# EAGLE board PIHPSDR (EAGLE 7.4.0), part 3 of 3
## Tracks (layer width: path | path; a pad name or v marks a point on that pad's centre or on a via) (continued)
N$1188  (via drill 0.8 pad 1.93) (continued)
  other vias: 151.94,107.22
N$1189  (via drill 0.8 pad 1.93)
  other vias: 151.94,104.68
N$1190  (via drill 0.8 pad 1.93)
  other vias: 151.94,102.14
N$1191  (via drill 0.8 pad 1.93)
  other vias: 151.94,99.6
N$1192  (via drill 0.8 pad 1.93)
  other vias: 151.94,97.06
N$1193  (via drill 0.8 pad 1.93)
  other vias: 151.94,94.52
N$1194  (via drill 0.8 pad 1.93)
  other vias: 151.94,91.98
N$1195  (via drill 0.8 pad 1.93)
  other vias: 151.94,89.44
N$1196  (via drill 0.8 pad 1.93)
  other vias: 151.94,86.9
N$1197  (via drill 0.8 pad 1.93)
  other vias: 151.94,84.36
N$1198  (via drill 0.8 pad 1.93)
  other vias: 151.94,81.82
N$1199  (via drill 0.8 pad 1.93)
  other vias: 151.94,79.28
N$1200  (via drill 0.8 pad 1.93)
  other vias: 151.94,76.74
N$1201  (via drill 0.8 pad 1.93)
  other vias: 151.94,74.2
N$1202  (via drill 0.8 pad 1.93)
  other vias: 151.94,71.66
N$1203  (via drill 0.8 pad 1.93)
  other vias: 151.94,69.12
N$1204  (via drill 0.8 pad 1.93)
  other vias: 151.94,66.58
N$1205  (via drill 0.8 pad 1.93)
  other vias: 151.94,64.04
N$1206  (via drill 0.8 pad 1.93)
  other vias: 151.94,61.5
N$1207  (via drill 0.8 pad 1.93)
  other vias: 151.94,58.96
N$1208  (via drill 0.8 pad 1.93)
  other vias: 151.94,56.42
N$1209  (via drill 0.8 pad 1.93)
  other vias: 151.94,53.88
N$1210  (via drill 0.8 pad 1.93)
  other vias: 151.94,51.34
N$1211  (via drill 0.8 pad 1.93)
  other vias: 151.94,48.8
N$1212  (via drill 0.8 pad 1.93)
  other vias: 151.94,46.26
N$1213  (via drill 0.8 pad 1.93)
  other vias: 151.94,43.72
N$1214  (via drill 0.8 pad 1.93)
  other vias: 151.94,41.18
N$1215  (via drill 0.8 pad 1.93)
  other vias: 151.94,38.64
N$1216  (via drill 0.8 pad 1.93)
  other vias: 151.94,36.1
N$1217  (via drill 0.8 pad 1.93)
  other vias: 151.94,33.56
N$1218  (via drill 0.8 pad 1.93)
  other vias: 151.94,31.02
N$1219  (via drill 0.8 pad 1.93)
  other vias: 151.94,28.48
N$1220  (via drill 0.8 pad 1.93)
  other vias: 151.94,25.94
N$1222  (via drill 0.8 pad 1.93)
  other vias: 154.48,119.92
N$1223  (via drill 0.8 pad 1.93)
  other vias: 154.48,117.38
N$1224  (via drill 0.8 pad 1.93)
  other vias: 154.48,114.84
N$1225  (via drill 0.8 pad 1.93)
  other vias: 154.48,112.3
N$1226  (via drill 0.8 pad 1.93)
  other vias: 154.48,109.76
N$1227  (via drill 0.8 pad 1.93)
  other vias: 154.48,107.22
N$1228  (via drill 0.8 pad 1.93)
  other vias: 154.48,104.68
N$1229  (via drill 0.8 pad 1.93)
  other vias: 154.48,102.14
N$1230  (via drill 0.8 pad 1.93)
  other vias: 154.48,99.6
N$1231  (via drill 0.8 pad 1.93)
  other vias: 154.48,97.06
N$1232  (via drill 0.8 pad 1.93)
  other vias: 154.48,94.52
N$1233  (via drill 0.8 pad 1.93)
  other vias: 154.48,91.98
N$1234  (via drill 0.8 pad 1.93)
  other vias: 154.48,89.44
N$1235  (via drill 0.8 pad 1.93)
  other vias: 154.48,86.9
N$1236  (via drill 0.8 pad 1.93)
  other vias: 154.48,84.36
N$1237  (via drill 0.8 pad 1.93)
  other vias: 154.48,81.82
N$1238  (via drill 0.8 pad 1.93)
  other vias: 154.48,79.28
N$1239  (via drill 0.8 pad 1.93)
  other vias: 154.48,76.74
N$1240  (via drill 0.8 pad 1.93)
  other vias: 154.48,74.2
N$1241  (via drill 0.8 pad 1.93)
  other vias: 154.48,71.66
N$1242  (via drill 0.8 pad 1.93)
  other vias: 154.48,69.12
N$1243  (via drill 0.8 pad 1.93)
  other vias: 154.48,66.58
N$1244  (via drill 0.8 pad 1.93)
  other vias: 154.48,64.04
N$1245  (via drill 0.8 pad 1.93)
  other vias: 154.48,61.5
N$1246  (via drill 0.8 pad 1.93)
  other vias: 154.48,58.96
N$1247  (via drill 0.8 pad 1.93)
  other vias: 154.48,56.42
N$1248  (via drill 0.8 pad 1.93)
  other vias: 154.48,53.88
N$1249  (via drill 0.8 pad 1.93)
  other vias: 154.48,51.34
N$1250  (via drill 0.8 pad 1.93)
  other vias: 154.48,48.8
N$1251  (via drill 0.8 pad 1.93)
  other vias: 154.48,46.26
N$1252  (via drill 0.8 pad 1.93)
  other vias: 154.48,43.72
N$1253  (via drill 0.8 pad 1.93)
  other vias: 154.48,41.18
N$1254  (via drill 0.8 pad 1.93)
  other vias: 154.48,38.64
N$1255  (via drill 0.8 pad 1.93)
  other vias: 154.48,36.1
N$1256  (via drill 0.8 pad 1.93)
  other vias: 154.48,33.56
N$1257  (via drill 0.8 pad 1.93)
  other vias: 154.48,31.02
N$1258  (via drill 0.8 pad 1.93)
  other vias: 154.48,28.48
N$1259  (via drill 0.8 pad 1.93)
  other vias: 154.48,25.94
N$1261  (via drill 0.8 pad 1.93)
  other vias: 157.02,119.92
N$1262  (via drill 0.8 pad 1.93)
  other vias: 157.02,117.38
N$1263  (via drill 0.8 pad 1.93)
  other vias: 157.02,114.84
N$1264  (via drill 0.8 pad 1.93)
  other vias: 157.02,112.3
N$1265  (via drill 0.8 pad 1.93)
  other vias: 157.02,109.76
N$1266  (via drill 0.8 pad 1.93)
  other vias: 157.02,107.22
N$1267  (via drill 0.8 pad 1.93)
  other vias: 157.02,104.68
N$1268  (via drill 0.8 pad 1.93)
  other vias: 157.02,102.14
N$1269  (via drill 0.8 pad 1.93)
  other vias: 157.02,99.6
N$1270  (via drill 0.8 pad 1.93)
  other vias: 157.02,97.06
N$1271  (via drill 0.8 pad 1.93)
  other vias: 157.02,94.52
N$1272  (via drill 0.8 pad 1.93)
  other vias: 157.02,91.98
N$1273  (via drill 0.8 pad 1.93)
  other vias: 157.02,89.44
N$1274  (via drill 0.8 pad 1.93)
  other vias: 157.02,86.9
N$1275  (via drill 0.8 pad 1.93)
  other vias: 157.02,84.36
N$1276  (via drill 0.8 pad 1.93)
  other vias: 157.02,81.82
N$1277  (via drill 0.8 pad 1.93)
  other vias: 157.02,79.28
N$1278  (via drill 0.8 pad 1.93)
  other vias: 157.02,76.74
N$1279  (via drill 0.8 pad 1.93)
  other vias: 157.02,74.2
N$1280  (via drill 0.8 pad 1.93)
  other vias: 157.02,71.66
N$1281  (via drill 0.8 pad 1.93)
  other vias: 157.02,69.12
N$1282  (via drill 0.8 pad 1.93)
  other vias: 157.02,66.58
N$1283  (via drill 0.8 pad 1.93)
  other vias: 157.02,64.04
N$1284  (via drill 0.8 pad 1.93)
  other vias: 157.02,61.5
N$1285  (via drill 0.8 pad 1.93)
  other vias: 157.02,58.96
N$1286  (via drill 0.8 pad 1.93)
  other vias: 157.02,56.42
N$1287  (via drill 0.8 pad 1.93)
  other vias: 157.02,53.88
N$1288  (via drill 0.8 pad 1.93)
  other vias: 157.02,51.34
N$1289  (via drill 0.8 pad 1.93)
  other vias: 157.02,48.8
N$1290  (via drill 0.8 pad 1.93)
  other vias: 157.02,46.26
N$1291  (via drill 0.8 pad 1.93)
  other vias: 157.02,43.72
N$1292  (via drill 0.8 pad 1.93)
  other vias: 157.02,41.18
N$1293  (via drill 0.8 pad 1.93)
  other vias: 157.02,38.64
N$1294  (via drill 0.8 pad 1.93)
  other vias: 157.02,36.1
N$1295  (via drill 0.8 pad 1.93)
  other vias: 157.02,33.56
N$1296  (via drill 0.8 pad 1.93)
  other vias: 157.02,31.02
N$1297  (via drill 0.8 pad 1.93)
  other vias: 157.02,28.48
N$1298  (via drill 0.8 pad 1.93)
  other vias: 157.02,25.94
N$1300  (via drill 0.8 pad 1.93)
  other vias: 159.56,119.92
N$1301  (via drill 0.8 pad 1.93)
  other vias: 159.56,117.38
N$1302  (via drill 0.8 pad 1.93)
  other vias: 159.56,114.84
N$1303  (via drill 0.8 pad 1.93)
  other vias: 159.56,112.3
N$1304  (via drill 0.8 pad 1.93)
  other vias: 159.56,109.76
N$1305  (via drill 0.8 pad 1.93)
  other vias: 159.56,107.22
N$1306  (via drill 0.8 pad 1.93)
  other vias: 159.56,104.68
N$1307  (via drill 0.8 pad 1.93)
  other vias: 159.56,102.14
N$1308  (via drill 0.8 pad 1.93)
  other vias: 159.56,99.6
N$1309  (via drill 0.8 pad 1.93)
  other vias: 159.56,97.06
N$1310  (via drill 0.8 pad 1.93)
  other vias: 159.56,94.52
N$1311  (via drill 0.8 pad 1.93)
  other vias: 159.56,91.98
N$1312  (via drill 0.8 pad 1.93)
  other vias: 159.56,89.44
N$1313  (via drill 0.8 pad 1.93)
  other vias: 159.56,86.9
N$1314  (via drill 0.8 pad 1.93)
  other vias: 159.56,84.36
N$1315  (via drill 0.8 pad 1.93)
  other vias: 159.56,81.82
N$1316  (via drill 0.8 pad 1.93)
  other vias: 159.56,79.28
N$1317  (via drill 0.8 pad 1.93)
  other vias: 159.56,76.74
N$1318  (via drill 0.8 pad 1.93)
  other vias: 159.56,74.2
N$1319  (via drill 0.8 pad 1.93)
  other vias: 159.56,71.66
N$1320  (via drill 0.8 pad 1.93)
  other vias: 159.56,69.12
N$1321  (via drill 0.8 pad 1.93)
  other vias: 159.56,66.58
N$1322  (via drill 0.8 pad 1.93)
  other vias: 159.56,64.04
N$1323  (via drill 0.8 pad 1.93)
  other vias: 159.56,61.5
N$1324  (via drill 0.8 pad 1.93)
  other vias: 159.56,58.96
N$1325  (via drill 0.8 pad 1.93)
  other vias: 159.56,56.42
N$1326  (via drill 0.8 pad 1.93)
  other vias: 159.56,53.88
N$1327  (via drill 0.8 pad 1.93)
  other vias: 159.56,51.34
N$1328  (via drill 0.8 pad 1.93)
  other vias: 159.56,48.8
N$1329  (via drill 0.8 pad 1.93)
  other vias: 159.56,46.26
N$1330  (via drill 0.8 pad 1.93)
  other vias: 159.56,43.72
N$1331  (via drill 0.8 pad 1.93)
  other vias: 159.56,41.18
N$1332  (via drill 0.8 pad 1.93)
  other vias: 159.56,38.64
N$1333  (via drill 0.8 pad 1.93)
  other vias: 159.56,36.1
N$1334  (via drill 0.8 pad 1.93)
  other vias: 159.56,33.56
N$1335  (via drill 0.8 pad 1.93)
  other vias: 159.56,31.02
N$1336  (via drill 0.8 pad 1.93)
  other vias: 159.56,28.48
N$1337  (via drill 0.8 pad 1.93)
  other vias: 159.56,25.94
N$1339  (via drill 0.8 pad 1.93)
  other vias: 162.1,119.92
N$1340  (via drill 0.8 pad 1.93)
  other vias: 162.1,117.38
N$1341  (via drill 0.8 pad 1.93)
  other vias: 162.1,114.84
N$1342  (via drill 0.8 pad 1.93)
  other vias: 162.1,112.3
N$1343  (via drill 0.8 pad 1.93)
  other vias: 162.1,109.76
N$1344  (via drill 0.8 pad 1.93)
  other vias: 162.1,107.22
N$1345  (via drill 0.8 pad 1.93)
  other vias: 162.1,104.68
N$1346  (via drill 0.8 pad 1.93)
  other vias: 162.1,102.14
N$1347  (via drill 0.8 pad 1.93)
  other vias: 162.1,99.6
N$1348  (via drill 0.8 pad 1.93)
  other vias: 162.1,97.06
N$1349  (via drill 0.8 pad 1.93)
  other vias: 162.1,94.52
N$1350  (via drill 0.8 pad 1.93)
  other vias: 162.1,91.98
N$1351  (via drill 0.8 pad 1.93)
  other vias: 162.1,89.44
N$1352  (via drill 0.8 pad 1.93)
  other vias: 162.1,86.9
N$1353  (via drill 0.8 pad 1.93)
  other vias: 162.1,84.36
N$1354  (via drill 0.8 pad 1.93)
  other vias: 162.1,81.82
N$1355  (via drill 0.8 pad 1.93)
  other vias: 162.1,79.28
N$1356  (via drill 0.8 pad 1.93)
  other vias: 162.1,76.74
N$1357  (via drill 0.8 pad 1.93)
  other vias: 162.1,74.2
N$1358  (via drill 0.8 pad 1.93)
  other vias: 162.1,71.66
N$1359  (via drill 0.8 pad 1.93)
  other vias: 162.1,69.12
N$1360  (via drill 0.8 pad 1.93)
  other vias: 162.1,66.58
N$1361  (via drill 0.8 pad 1.93)
  other vias: 162.1,64.04
N$1362  (via drill 0.8 pad 1.93)
  other vias: 162.1,61.5
N$1363  (via drill 0.8 pad 1.93)
  other vias: 162.1,58.96
N$1364  (via drill 0.8 pad 1.93)
  other vias: 162.1,56.42
N$1365  (via drill 0.8 pad 1.93)
  other vias: 162.1,53.88
N$1366  (via drill 0.8 pad 1.93)
  other vias: 162.1,51.34
N$1367  (via drill 0.8 pad 1.93)
  other vias: 162.1,48.8
N$1368  (via drill 0.8 pad 1.93)
  other vias: 162.1,46.26
N$1369  (via drill 0.8 pad 1.93)
  other vias: 162.1,43.72
N$1370  (via drill 0.8 pad 1.93)
  other vias: 162.1,41.18
N$1371  (via drill 0.8 pad 1.93)
  other vias: 162.1,38.64
N$1372  (via drill 0.8 pad 1.93)
  other vias: 162.1,36.1
N$1373  (via drill 0.8 pad 1.93)
  other vias: 162.1,33.56
N$1374  (via drill 0.8 pad 1.93)
  other vias: 162.1,31.02
N$1375  (via drill 0.8 pad 1.93)
  other vias: 162.1,28.48
N$1376  (via drill 0.8 pad 1.93)
  other vias: 162.1,25.94
N$1378  (via drill 0.8 pad 1.93)
  other vias: 164.64,119.92
N$1379  (via drill 0.8 pad 1.93)
  other vias: 164.64,117.38
N$1380  (via drill 0.8 pad 1.93)
  other vias: 164.64,114.84
N$1381  (via drill 0.8 pad 1.93)
  other vias: 164.64,112.3
N$1382  (via drill 0.8 pad 1.93)
  other vias: 164.64,109.76
N$1383  (via drill 0.8 pad 1.93)
  other vias: 164.64,107.22
N$1384  (via drill 0.8 pad 1.93)
  other vias: 164.64,104.68
N$1385  (via drill 0.8 pad 1.93)
  other vias: 164.64,102.14
N$1386  (via drill 0.8 pad 1.93)
  other vias: 164.64,99.6
N$1387  (via drill 0.8 pad 1.93)
  other vias: 164.64,97.06
N$1388  (via drill 0.8 pad 1.93)
  other vias: 164.64,94.52
N$1389  (via drill 0.8 pad 1.93)
  other vias: 164.64,91.98
N$1390  (via drill 0.8 pad 1.93)
  other vias: 164.64,89.44
N$1391  (via drill 0.8 pad 1.93)
  other vias: 164.64,86.9
N$1392  (via drill 0.8 pad 1.93)
  other vias: 164.64,84.36
N$1393  (via drill 0.8 pad 1.93)
  other vias: 164.64,81.82
N$1394  (via drill 0.8 pad 1.93)
  other vias: 164.64,79.28
N$1395  (via drill 0.8 pad 1.93)
  other vias: 164.64,76.74
N$1396  (via drill 0.8 pad 1.93)
  other vias: 164.64,74.2
N$1397  (via drill 0.8 pad 1.93)
  other vias: 164.64,71.66
N$1398  (via drill 0.8 pad 1.93)
  other vias: 164.64,69.12
N$1399  (via drill 0.8 pad 1.93)
  other vias: 164.64,66.58
N$1400  (via drill 0.8 pad 1.93)
  other vias: 164.64,64.04
N$1401  (via drill 0.8 pad 1.93)
  other vias: 164.64,61.5
N$1402  (via drill 0.8 pad 1.93)
  other vias: 164.64,58.96
N$1403  (via drill 0.8 pad 1.93)
  other vias: 164.64,56.42
N$1404  (via drill 0.8 pad 1.93)
  other vias: 164.64,53.88
N$1405  (via drill 0.8 pad 1.93)
  other vias: 164.64,51.34
N$1406  (via drill 0.8 pad 1.93)
  other vias: 164.64,48.8
N$1407  (via drill 0.8 pad 1.93)
  other vias: 164.64,46.26
N$1408  (via drill 0.8 pad 1.93)
  other vias: 164.64,43.72
N$1409  (via drill 0.8 pad 1.93)
  other vias: 164.64,41.18
N$1410  (via drill 0.8 pad 1.93)
  other vias: 164.64,38.64
N$1411  (via drill 0.8 pad 1.93)
  other vias: 164.64,36.1
N$1412  (via drill 0.8 pad 1.93)
  other vias: 164.64,33.56
N$1413  (via drill 0.8 pad 1.93)
  other vias: 164.64,31.02
N$1414  (via drill 0.8 pad 1.93)
  other vias: 164.64,28.48
N$1415  (via drill 0.8 pad 1.93)
  other vias: 164.64,25.94
N$1417  (via drill 0.8 pad 1.93)
  other vias: 167.18,119.92
N$1418  (via drill 0.8 pad 1.93)
  other vias: 167.18,117.38
N$1419  (via drill 0.8 pad 1.93)
  other vias: 167.18,114.84
N$1420  (via drill 0.8 pad 1.93)
  other vias: 167.18,112.3
N$1421  (via drill 0.8 pad 1.93)
  other vias: 167.18,109.76
N$1422  (via drill 0.8 pad 1.93)
  other vias: 167.18,107.22
N$1423  (via drill 0.8 pad 1.93)
  other vias: 167.18,104.68
N$1424  (via drill 0.8 pad 1.93)
  other vias: 167.18,102.14
N$1425  (via drill 0.8 pad 1.93)
  other vias: 167.18,99.6
N$1426  (via drill 0.8 pad 1.93)
  other vias: 167.18,97.06
N$1427  (via drill 0.8 pad 1.93)
  other vias: 167.18,94.52
N$1428  (via drill 0.8 pad 1.93)
  other vias: 167.18,91.98
N$1429  (via drill 0.8 pad 1.93)
  other vias: 167.18,89.44
N$1430  (via drill 0.8 pad 1.93)
  other vias: 167.18,86.9
N$1431  (via drill 0.8 pad 1.93)
  other vias: 167.18,84.36
N$1432  (via drill 0.8 pad 1.93)
  other vias: 167.18,81.82
N$1433  (via drill 0.8 pad 1.93)
  other vias: 167.18,79.28
N$1434  (via drill 0.8 pad 1.93)
  other vias: 167.18,76.74
N$1435  (via drill 0.8 pad 1.93)
  other vias: 167.18,74.2
N$1436  (via drill 0.8 pad 1.93)
  other vias: 167.18,71.66
N$1437  (via drill 0.8 pad 1.93)
  other vias: 167.18,69.12
N$1438  (via drill 0.8 pad 1.93)
  other vias: 167.18,66.58
N$1439  (via drill 0.8 pad 1.93)
  other vias: 167.18,64.04
N$1440  (via drill 0.8 pad 1.93)
  other vias: 167.18,61.5
N$1441  (via drill 0.8 pad 1.93)
  other vias: 167.18,58.96
N$1442  (via drill 0.8 pad 1.93)
  other vias: 167.18,56.42
N$1443  (via drill 0.8 pad 1.93)
  other vias: 167.18,53.88
N$1444  (via drill 0.8 pad 1.93)
  other vias: 167.18,51.34
N$1445  (via drill 0.8 pad 1.93)
  other vias: 167.18,48.8
N$1446  (via drill 0.8 pad 1.93)
  other vias: 167.18,46.26
N$1447  (via drill 0.8 pad 1.93)
  other vias: 167.18,43.72
N$1448  (via drill 0.8 pad 1.93)
  other vias: 167.18,41.18
N$1449  (via drill 0.8 pad 1.93)
  other vias: 167.18,38.64
N$1450  (via drill 0.8 pad 1.93)
  other vias: 167.18,36.1
N$1451  (via drill 0.8 pad 1.93)
  other vias: 167.18,33.56
N$1452  (via drill 0.8 pad 1.93)
  other vias: 167.18,31.02
N$1453  (via drill 0.8 pad 1.93)
  other vias: 167.18,28.48
N$1454  (via drill 0.8 pad 1.93)
  other vias: 167.18,25.94
N$1456  (via drill 0.8 pad 1.93)
  other vias: 172.26,119.92
N$1457  (via drill 0.8 pad 1.93)
  other vias: 172.26,117.38
N$1458  (via drill 0.8 pad 1.93)
  other vias: 172.26,114.84
N$1459  (via drill 0.8 pad 1.93)
  other vias: 172.26,112.3
N$1460  (via drill 0.8 pad 1.93)
  other vias: 172.26,109.76
N$1461  (via drill 0.8 pad 1.93)
  other vias: 172.26,107.22
N$1462  (via drill 0.8 pad 1.93)
  other vias: 172.26,104.68
N$1463  (via drill 0.8 pad 1.93)
  other vias: 172.26,102.14
N$1464  (via drill 0.8 pad 1.93)
  other vias: 172.26,99.6
N$1465  (via drill 0.8 pad 1.93)
  other vias: 172.26,97.06
N$1466  (via drill 0.8 pad 1.93)
  other vias: 172.26,94.52
N$1467  (via drill 0.8 pad 1.93)
  other vias: 172.26,91.98
N$1468  (via drill 0.8 pad 1.93)
  other vias: 172.26,89.44
N$1469  (via drill 0.8 pad 1.93)
  other vias: 172.26,86.9
N$1470  (via drill 0.8 pad 1.93)
  other vias: 172.26,84.36
N$1471  (via drill 0.8 pad 1.93)
  other vias: 172.26,81.82
N$1472  (via drill 0.8 pad 1.93)
  other vias: 172.26,79.28
N$1473  (via drill 0.8 pad 1.93)
  other vias: 172.26,76.74
N$1474  (via drill 0.8 pad 1.93)
  other vias: 172.26,74.2
N$1475  (via drill 0.8 pad 1.93)
  other vias: 172.26,71.66
N$1476  (via drill 0.8 pad 1.93)
  other vias: 172.26,69.12
N$1477  (via drill 0.8 pad 1.93)
  other vias: 172.26,66.58
N$1478  (via drill 0.8 pad 1.93)
  other vias: 172.26,64.04
N$1479  (via drill 0.8 pad 1.93)
  other vias: 172.26,61.5
N$1480  (via drill 0.8 pad 1.93)
  other vias: 172.26,58.96
N$1481  (via drill 0.8 pad 1.93)
  other vias: 172.26,56.42
N$1482  (via drill 0.8 pad 1.93)
  other vias: 172.26,53.88
N$1483  (via drill 0.8 pad 1.93)
  other vias: 172.26,51.34
N$1484  (via drill 0.8 pad 1.93)
  other vias: 172.26,48.8
N$1485  (via drill 0.8 pad 1.93)
  other vias: 172.26,46.26
N$1486  (via drill 0.8 pad 1.93)
  other vias: 172.26,43.72
N$1487  (via drill 0.8 pad 1.93)
  other vias: 172.26,41.18
N$1488  (via drill 0.8 pad 1.93)
  other vias: 172.26,38.64
N$1489  (via drill 0.8 pad 1.93)
  other vias: 172.26,36.1
N$1490  (via drill 0.8 pad 1.93)
  other vias: 172.26,33.56
N$1491  (via drill 0.8 pad 1.93)
  other vias: 172.26,31.02
N$1492  (via drill 0.8 pad 1.93)
  other vias: 172.26,28.48
N$1493  (via drill 0.8 pad 1.93)
  other vias: 172.26,25.94
N$1495  (via drill 0.8 pad 1.93)
  other vias: 169.72,119.92
N$1496  (via drill 0.8 pad 1.93)
  other vias: 169.72,117.38
N$1497  (via drill 0.8 pad 1.93)
  other vias: 169.72,114.84
N$1498  (via drill 0.8 pad 1.93)
  other vias: 169.72,112.3
N$1499  (via drill 0.8 pad 1.93)
  other vias: 169.72,109.76
N$1500  (via drill 0.8 pad 1.93)
  other vias: 169.72,107.22
N$1501  (via drill 0.8 pad 1.93)
  other vias: 169.72,104.68
N$1502  (via drill 0.8 pad 1.93)
  other vias: 169.72,102.14
N$1503  (via drill 0.8 pad 1.93)
  other vias: 169.72,99.6
N$1504  (via drill 0.8 pad 1.93)
  other vias: 169.72,97.06
N$1505  (via drill 0.8 pad 1.93)
  other vias: 169.72,94.52
N$1506  (via drill 0.8 pad 1.93)
  other vias: 169.72,91.98
N$1507  (via drill 0.8 pad 1.93)
  other vias: 169.72,89.44
N$1508  (via drill 0.8 pad 1.93)
  other vias: 169.72,86.9
N$1509  (via drill 0.8 pad 1.93)
  other vias: 169.72,84.36
N$1510  (via drill 0.8 pad 1.93)
  other vias: 169.72,81.82
N$1511  (via drill 0.8 pad 1.93)
  other vias: 169.72,79.28
N$1512  (via drill 0.8 pad 1.93)
  other vias: 169.72,76.74
N$1513  (via drill 0.8 pad 1.93)
  other vias: 169.72,74.2
N$1514  (via drill 0.8 pad 1.93)
  other vias: 169.72,71.66
N$1515  (via drill 0.8 pad 1.93)
  other vias: 169.72,69.12
N$1516  (via drill 0.8 pad 1.93)
  other vias: 169.72,66.58
N$1517  (via drill 0.8 pad 1.93)
  other vias: 169.72,64.04
N$1518  (via drill 0.8 pad 1.93)
  other vias: 169.72,61.5
N$1519  (via drill 0.8 pad 1.93)
  other vias: 169.72,58.96
N$1520  (via drill 0.8 pad 1.93)
  other vias: 169.72,56.42
N$1521  (via drill 0.8 pad 1.93)
  other vias: 169.72,53.88
N$1522  (via drill 0.8 pad 1.93)
  other vias: 169.72,51.34
N$1523  (via drill 0.8 pad 1.93)
  other vias: 169.72,48.8
N$1524  (via drill 0.8 pad 1.93)
  other vias: 169.72,46.26
N$1525  (via drill 0.8 pad 1.93)
  other vias: 169.72,43.72
N$1526  (via drill 0.8 pad 1.93)
  other vias: 169.72,41.18
N$1527  (via drill 0.8 pad 1.93)
  other vias: 169.72,38.64
N$1528  (via drill 0.8 pad 1.93)
  other vias: 169.72,36.1
N$1529  (via drill 0.8 pad 1.93)
  other vias: 169.72,33.56
N$1530  (via drill 0.8 pad 1.93)
  other vias: 169.72,31.02
N$1531  (via drill 0.8 pad 1.93)
  other vias: 169.72,28.48
N$1532  (via drill 0.8 pad 1.93)
  other vias: 169.72,25.94
N$1534  (via drill 0.8 pad 1.93)
  other vias: 174.8,119.92
N$1535  (via drill 0.8 pad 1.93)
  other vias: 174.8,117.38
N$1536  (via drill 0.8 pad 1.93)
  other vias: 174.8,114.84
N$1537  (via drill 0.8 pad 1.93)
  other vias: 174.8,112.3
N$1538  (via drill 0.8 pad 1.93)
  other vias: 174.8,109.76
N$1539  (via drill 0.8 pad 1.93)
  other vias: 174.8,107.22
N$1540  (via drill 0.8 pad 1.93)
  other vias: 174.8,104.68
N$1541  (via drill 0.8 pad 1.93)
  other vias: 174.8,102.14
N$1542  (via drill 0.8 pad 1.93)
  other vias: 174.8,99.6
N$1543  (via drill 0.8 pad 1.93)
  other vias: 174.8,97.06
N$1544  (via drill 0.8 pad 1.93)
  other vias: 174.8,94.52
N$1545  (via drill 0.8 pad 1.93)
  other vias: 174.8,91.98
N$1546  (via drill 0.8 pad 1.93)
  other vias: 174.8,89.44
N$1547  (via drill 0.8 pad 1.93)
  other vias: 174.8,86.9
N$1548  (via drill 0.8 pad 1.93)
  other vias: 174.8,84.36
N$1549  (via drill 0.8 pad 1.93)
  other vias: 174.8,81.82
N$1550  (via drill 0.8 pad 1.93)
  other vias: 174.8,79.28
N$1551  (via drill 0.8 pad 1.93)
  other vias: 174.8,76.74
N$1552  (via drill 0.8 pad 1.93)
  other vias: 174.8,74.2
N$1553  (via drill 0.8 pad 1.93)
  other vias: 174.8,71.66
N$1554  (via drill 0.8 pad 1.93)
  other vias: 174.8,69.12
N$1555  (via drill 0.8 pad 1.93)
  other vias: 174.8,66.58
N$1556  (via drill 0.8 pad 1.93)
  other vias: 174.8,64.04
N$1557  (via drill 0.8 pad 1.93)
  other vias: 174.8,61.5
N$1558  (via drill 0.8 pad 1.93)
  other vias: 174.8,58.96
N$1559  (via drill 0.8 pad 1.93)
  other vias: 174.8,56.42
N$1560  (via drill 0.8 pad 1.93)
  other vias: 174.8,53.88
N$1561  (via drill 0.8 pad 1.93)
  other vias: 174.8,51.34
N$1562  (via drill 0.8 pad 1.93)
  other vias: 174.8,48.8
N$1563  (via drill 0.8 pad 1.93)
  other vias: 174.8,46.26
N$1564  (via drill 0.8 pad 1.93)
  other vias: 174.8,43.72
N$1565  (via drill 0.8 pad 1.93)
  other vias: 174.8,41.18
N$1566  (via drill 0.8 pad 1.93)
  other vias: 174.8,38.64
N$1567  (via drill 0.8 pad 1.93)
  other vias: 174.8,36.1
N$1568  (via drill 0.8 pad 1.93)
  other vias: 174.8,33.56
N$1569  (via drill 0.8 pad 1.93)
  other vias: 174.8,31.02
N$1570  (via drill 0.8 pad 1.93)
  other vias: 174.8,28.48
N$1571  (via drill 0.8 pad 1.93)
  other vias: 174.8,25.94
N$1573  (via drill 0.8 pad 1.93)
  other vias: 177.34,119.92
N$1574  (via drill 0.8 pad 1.93)
  other vias: 177.34,117.38
N$1575  (via drill 0.8 pad 1.93)
  other vias: 177.34,114.84
N$1576  (via drill 0.8 pad 1.93)
  other vias: 177.34,112.3
N$1577  (via drill 0.8 pad 1.93)
  other vias: 177.34,109.76
N$1578  (via drill 0.8 pad 1.93)
  other vias: 177.34,107.22
N$1579  (via drill 0.8 pad 1.93)
  other vias: 177.34,104.68
N$1580  (via drill 0.8 pad 1.93)
  other vias: 177.34,102.14
N$1581  (via drill 0.8 pad 1.93)
  other vias: 177.34,99.6
N$1582  (via drill 0.8 pad 1.93)
  other vias: 177.34,97.06
N$1583  (via drill 0.8 pad 1.93)
  other vias: 177.34,94.52
N$1584  (via drill 0.8 pad 1.93)
  other vias: 177.34,91.98
N$1585  (via drill 0.8 pad 1.93)
  other vias: 177.34,89.44
N$1586  (via drill 0.8 pad 1.93)
  other vias: 177.34,86.9
N$1587  (via drill 0.8 pad 1.93)
  other vias: 177.34,84.36
N$1588  (via drill 0.8 pad 1.93)
  other vias: 177.34,81.82
N$1589  (via drill 0.8 pad 1.93)
  other vias: 177.34,79.28
N$1590  (via drill 0.8 pad 1.93)
  other vias: 177.34,76.74
N$1591  (via drill 0.8 pad 1.93)
  other vias: 177.34,74.2
N$1592  (via drill 0.8 pad 1.93)
  other vias: 177.34,71.66
N$1593  (via drill 0.8 pad 1.93)
  other vias: 177.34,69.12
N$1594  (via drill 0.8 pad 1.93)
  other vias: 177.34,66.58
N$1595  (via drill 0.8 pad 1.93)
  other vias: 177.34,64.04
N$1596  (via drill 0.8 pad 1.93)
  other vias: 177.34,61.5
N$1597  (via drill 0.8 pad 1.93)
  other vias: 177.34,58.96
N$1598  (via drill 0.8 pad 1.93)
  other vias: 177.34,56.42
N$1599  (via drill 0.8 pad 1.93)
  other vias: 177.34,53.88
N$1600  (via drill 0.8 pad 1.93)
  other vias: 177.34,51.34
N$1601  (via drill 0.8 pad 1.93)
  other vias: 177.34,48.8
N$1602  (via drill 0.8 pad 1.93)
  other vias: 177.34,46.26
N$1603  (via drill 0.8 pad 1.93)
  other vias: 177.34,43.72
N$1604  (via drill 0.8 pad 1.93)
  other vias: 177.34,41.18
N$1605  (via drill 0.8 pad 1.93)
  other vias: 177.34,38.64
N$1606  (via drill 0.8 pad 1.93)
  other vias: 177.34,36.1
N$1607  (via drill 0.8 pad 1.93)
  other vias: 177.34,33.56
N$1608  (via drill 0.8 pad 1.93)
  other vias: 177.34,31.02
N$1609  (via drill 0.8 pad 1.93)
  other vias: 177.34,28.48
N$1610  (via drill 0.8 pad 1.93)
  other vias: 177.34,25.94
N$1612  (via drill 0.8 pad 1.93)
  other vias: 179.88,119.92
N$1613  (via drill 0.8 pad 1.93)
  other vias: 179.88,117.38
N$1614  (via drill 0.8 pad 1.93)
  other vias: 179.88,114.84
N$1615  (via drill 0.8 pad 1.93)
  other vias: 179.88,112.3
N$1616  (via drill 0.8 pad 1.93)
  other vias: 179.88,109.76
N$1617  (via drill 0.8 pad 1.93)
  other vias: 179.88,107.22
N$1618  (via drill 0.8 pad 1.93)
  other vias: 179.88,104.68
N$1619  (via drill 0.8 pad 1.93)
  other vias: 179.88,102.14
N$1620  (via drill 0.8 pad 1.93)
  other vias: 179.88,99.6
N$1621  (via drill 0.8 pad 1.93)
  other vias: 179.88,97.06
N$1622  (via drill 0.8 pad 1.93)
  other vias: 179.88,94.52
N$1623  (via drill 0.8 pad 1.93)
  other vias: 179.88,91.98
N$1624  (via drill 0.8 pad 1.93)
  other vias: 179.88,89.44
N$1625  (via drill 0.8 pad 1.93)
  other vias: 179.88,86.9
N$1626  (via drill 0.8 pad 1.93)
  other vias: 179.88,84.36
N$1627  (via drill 0.8 pad 1.93)
  other vias: 179.88,81.82
N$1628  (via drill 0.8 pad 1.93)
  other vias: 179.88,79.28
N$1629  (via drill 0.8 pad 1.93)
  other vias: 179.88,76.74
N$1630  (via drill 0.8 pad 1.93)
  other vias: 179.88,74.2
N$1631  (via drill 0.8 pad 1.93)
  other vias: 179.88,71.66
N$1632  (via drill 0.8 pad 1.93)
  other vias: 179.88,69.12
N$1633  (via drill 0.8 pad 1.93)
  other vias: 179.88,66.58
N$1634  (via drill 0.8 pad 1.93)
  other vias: 179.88,64.04
N$1635  (via drill 0.8 pad 1.93)
  other vias: 179.88,61.5
N$1636  (via drill 0.8 pad 1.93)
  other vias: 179.88,58.96
N$1637  (via drill 0.8 pad 1.93)
  other vias: 179.88,56.42
N$1638  (via drill 0.8 pad 1.93)
  other vias: 179.88,53.88
N$1639  (via drill 0.8 pad 1.93)
  other vias: 179.88,51.34
N$1640  (via drill 0.8 pad 1.93)
  other vias: 179.88,48.8
N$1641  (via drill 0.8 pad 1.93)
  other vias: 179.88,46.26
N$1642  (via drill 0.8 pad 1.93)
  other vias: 179.88,43.72
N$1643  (via drill 0.8 pad 1.93)
  other vias: 179.88,41.18
N$1644  (via drill 0.8 pad 1.93)
  other vias: 179.88,38.64
N$1645  (via drill 0.8 pad 1.93)
  other vias: 179.88,36.1
N$1646  (via drill 0.8 pad 1.93)
  other vias: 179.88,33.56
N$1647  (via drill 0.8 pad 1.93)
  other vias: 179.88,31.02
N$1648  (via drill 0.8 pad 1.93)
  other vias: 179.88,28.48
N$1649  (via drill 0.8 pad 1.93)
  other vias: 179.88,25.94
N$1651  (via drill 0.8 pad 1.93)
  other vias: 182.42,119.92
N$1652  (via drill 0.8 pad 1.93)
  other vias: 182.42,117.38
N$1653  (via drill 0.8 pad 1.93)
  other vias: 182.42,114.84
N$1654  (via drill 0.8 pad 1.93)
  other vias: 182.42,112.3
N$1655  (via drill 0.8 pad 1.93)
  other vias: 182.42,109.76
N$1656  (via drill 0.8 pad 1.93)
  other vias: 182.42,107.22
N$1657  (via drill 0.8 pad 1.93)
  other vias: 182.42,104.68
N$1658  (via drill 0.8 pad 1.93)
  other vias: 182.42,102.14
N$1659  (via drill 0.8 pad 1.93)
  other vias: 182.42,99.6
N$1660  (via drill 0.8 pad 1.93)
  other vias: 182.42,97.06
N$1661  (via drill 0.8 pad 1.93)
  other vias: 182.42,94.52
N$1662  (via drill 0.8 pad 1.93)
  other vias: 182.42,91.98
N$1663  (via drill 0.8 pad 1.93)
  other vias: 182.42,89.44
N$1664  (via drill 0.8 pad 1.93)
  other vias: 182.42,86.9
N$1665  (via drill 0.8 pad 1.93)
  other vias: 182.42,84.36
N$1666  (via drill 0.8 pad 1.93)
  other vias: 182.42,81.82
N$1667  (via drill 0.8 pad 1.93)
  other vias: 182.42,79.28
N$1668  (via drill 0.8 pad 1.93)
  other vias: 182.42,76.74
N$1669  (via drill 0.8 pad 1.93)
  other vias: 182.42,74.2
N$1670  (via drill 0.8 pad 1.93)
  other vias: 182.42,71.66
N$1671  (via drill 0.8 pad 1.93)
  other vias: 182.42,69.12
N$1672  (via drill 0.8 pad 1.93)
  other vias: 182.42,66.58
N$1673  (via drill 0.8 pad 1.93)
  other vias: 182.42,64.04
N$1674  (via drill 0.8 pad 1.93)
  other vias: 182.42,61.5
N$1675  (via drill 0.8 pad 1.93)
  other vias: 182.42,58.96
N$1676  (via drill 0.8 pad 1.93)
  other vias: 182.42,56.42
N$1677  (via drill 0.8 pad 1.93)
  other vias: 182.42,53.88
N$1678  (via drill 0.8 pad 1.93)
  other vias: 182.42,51.34
N$1679  (via drill 0.8 pad 1.93)
  other vias: 182.42,48.8
N$1680  (via drill 0.8 pad 1.93)
  other vias: 182.42,46.26
N$1681  (via drill 0.8 pad 1.93)
  other vias: 182.42,43.72
N$1682  (via drill 0.8 pad 1.93)
  other vias: 182.42,41.18
N$1683  (via drill 0.8 pad 1.93)
  other vias: 182.42,38.64
N$1684  (via drill 0.8 pad 1.93)
  other vias: 182.42,36.1
N$1685  (via drill 0.8 pad 1.93)
  other vias: 182.42,33.56
N$1686  (via drill 0.8 pad 1.93)
  other vias: 182.42,31.02
N$1687  (via drill 0.8 pad 1.93)
  other vias: 182.42,28.48
N$1688  (via drill 0.8 pad 1.93)
  other vias: 182.42,25.94
N$1690  (via drill 0.8 pad 1.93)
  other vias: 184.96,119.92
N$1691  (via drill 0.8 pad 1.93)
  other vias: 184.96,117.38
N$1692  (via drill 0.8 pad 1.93)
  other vias: 184.96,114.84
N$1693  (via drill 0.8 pad 1.93)
  other vias: 184.96,112.3
N$1694  (via drill 0.8 pad 1.93)
  other vias: 184.96,109.76
N$1695  (via drill 0.8 pad 1.93)
  other vias: 184.96,107.22
N$1696  (via drill 0.8 pad 1.93)
  other vias: 184.96,104.68
N$1697  (via drill 0.8 pad 1.93)
  other vias: 184.96,102.14
N$1698  (via drill 0.8 pad 1.93)
  other vias: 184.96,99.6
N$1699  (via drill 0.8 pad 1.93)
  other vias: 184.96,97.06
N$1700  (via drill 0.8 pad 1.93)
  other vias: 184.96,94.52
N$1701  (via drill 0.8 pad 1.93)
  other vias: 184.96,91.98
N$1702  (via drill 0.8 pad 1.93)
  other vias: 184.96,89.44
N$1703  (via drill 0.8 pad 1.93)
  other vias: 184.96,86.9
N$1704  (via drill 0.8 pad 1.93)
  other vias: 184.96,84.36
N$1705  (via drill 0.8 pad 1.93)
  other vias: 184.96,81.82
N$1706  (via drill 0.8 pad 1.93)
  other vias: 184.96,79.28
N$1707  (via drill 0.8 pad 1.93)
  other vias: 184.96,76.74
N$1708  (via drill 0.8 pad 1.93)
  other vias: 184.96,74.2
N$1709  (via drill 0.8 pad 1.93)
  other vias: 184.96,71.66
N$1710  (via drill 0.8 pad 1.93)
  other vias: 184.96,69.12
N$1711  (via drill 0.8 pad 1.93)
  other vias: 184.96,66.58
N$1712  (via drill 0.8 pad 1.93)
  other vias: 184.96,64.04
N$1713  (via drill 0.8 pad 1.93)
  other vias: 184.96,61.5
N$1714  (via drill 0.8 pad 1.93)
  other vias: 184.96,58.96
N$1715  (via drill 0.8 pad 1.93)
  other vias: 184.96,56.42
N$1716  (via drill 0.8 pad 1.93)
  other vias: 184.96,53.88
N$1717  (via drill 0.8 pad 1.93)
  other vias: 184.96,51.34
N$1718  (via drill 0.8 pad 1.93)
  other vias: 184.96,48.8
N$1719  (via drill 0.8 pad 1.93)
  other vias: 184.96,46.26
N$1720  (via drill 0.8 pad 1.93)
  other vias: 184.96,43.72
N$1721  (via drill 0.8 pad 1.93)
  other vias: 184.96,41.18
N$1722  (via drill 0.8 pad 1.93)
  other vias: 184.96,38.64
N$1723  (via drill 0.8 pad 1.93)
  other vias: 184.96,36.1
N$1724  (via drill 0.8 pad 1.93)
  other vias: 184.96,33.56
N$1725  (via drill 0.8 pad 1.93)
  other vias: 184.96,31.02
N$1726  (via drill 0.8 pad 1.93)
  other vias: 184.96,28.48
N$1727  (via drill 0.8 pad 1.93)
  other vias: 184.96,25.94
N$1729  (via drill 0.8 pad 1.93)
  other vias: 187.5,119.92
N$1730  (via drill 0.8 pad 1.93)
  other vias: 187.5,117.38
N$1731  (via drill 0.8 pad 1.93)
  other vias: 187.5,114.84
N$1732  (via drill 0.8 pad 1.93)
  other vias: 187.5,112.3
N$1733  (via drill 0.8 pad 1.93)
  other vias: 187.5,109.76
N$1734  (via drill 0.8 pad 1.93)
  other vias: 187.5,107.22
N$1735  (via drill 0.8 pad 1.93)
  other vias: 187.5,104.68
N$1736  (via drill 0.8 pad 1.93)
  other vias: 187.5,102.14
N$1737  (via drill 0.8 pad 1.93)
  other vias: 187.5,99.6
N$1738  (via drill 0.8 pad 1.93)
  other vias: 187.5,97.06
N$1739  (via drill 0.8 pad 1.93)
  other vias: 187.5,94.52
N$1740  (via drill 0.8 pad 1.93)
  other vias: 187.5,91.98
N$1741  (via drill 0.8 pad 1.93)
  other vias: 187.5,89.44
N$1742  (via drill 0.8 pad 1.93)
  other vias: 187.5,86.9
N$1743  (via drill 0.8 pad 1.93)
  other vias: 187.5,84.36
N$1744  (via drill 0.8 pad 1.93)
  other vias: 187.5,81.82
N$1745  (via drill 0.8 pad 1.93)
  other vias: 187.5,79.28
N$1746  (via drill 0.8 pad 1.93)
  other vias: 187.5,76.74
N$1747  (via drill 0.8 pad 1.93)
  other vias: 187.5,74.2
N$1748  (via drill 0.8 pad 1.93)
  other vias: 187.5,71.66
N$1749  (via drill 0.8 pad 1.93)
  other vias: 187.5,69.12
N$1750  (via drill 0.8 pad 1.93)
  other vias: 187.5,66.58
N$1751  (via drill 0.8 pad 1.93)
  other vias: 187.5,64.04
N$1752  (via drill 0.8 pad 1.93)
  other vias: 187.5,61.5
N$1753  (via drill 0.8 pad 1.93)
  other vias: 187.5,58.96
N$1754  (via drill 0.8 pad 1.93)
  other vias: 187.5,56.42
N$1755  (via drill 0.8 pad 1.93)
  other vias: 187.5,53.88
N$1756  (via drill 0.8 pad 1.93)
  other vias: 187.5,51.34
N$1757  (via drill 0.8 pad 1.93)
  other vias: 187.5,48.8
N$1758  (via drill 0.8 pad 1.93)
  other vias: 187.5,46.26
N$1759  (via drill 0.8 pad 1.93)
  other vias: 187.5,43.72
N$1760  (via drill 0.8 pad 1.93)
  other vias: 187.5,41.18
N$1761  (via drill 0.8 pad 1.93)
  other vias: 187.5,38.64
N$1762  (via drill 0.8 pad 1.93)
  other vias: 187.5,36.1
N$1763  (via drill 0.8 pad 1.93)
  other vias: 187.5,33.56
N$1764  (via drill 0.8 pad 1.93)
  other vias: 187.5,31.02
N$1765  (via drill 0.8 pad 1.93)
  other vias: 187.5,28.48
N$1766  (via drill 0.8 pad 1.93)
  other vias: 187.5,25.94
N$1768  (via drill 0.8 pad 1.93)
  other vias: 190.04,119.92
N$1769  (via drill 0.8 pad 1.93)
  other vias: 190.04,117.38
N$1770  (via drill 0.8 pad 1.93)
  other vias: 190.04,114.84
N$1771  (via drill 0.8 pad 1.93)
  other vias: 190.04,112.3
N$1772  (via drill 0.8 pad 1.93)
  other vias: 190.04,109.76
N$1773  (via drill 0.8 pad 1.93)
  other vias: 190.04,107.22
N$1774  (via drill 0.8 pad 1.93)
  other vias: 190.04,104.68
N$1775  (via drill 0.8 pad 1.93)
  other vias: 190.04,102.14
N$1776  (via drill 0.8 pad 1.93)
  other vias: 190.04,99.6
N$1777  (via drill 0.8 pad 1.93)
  other vias: 190.04,97.06
N$1778  (via drill 0.8 pad 1.93)
  other vias: 190.04,94.52
N$1779  (via drill 0.8 pad 1.93)
  other vias: 190.04,91.98
N$1780  (via drill 0.8 pad 1.93)
  other vias: 190.04,89.44
N$1781  (via drill 0.8 pad 1.93)
  other vias: 190.04,86.9
N$1782  (via drill 0.8 pad 1.93)
  other vias: 190.04,84.36
N$1783  (via drill 0.8 pad 1.93)
  other vias: 190.04,81.82
N$1784  (via drill 0.8 pad 1.93)
  other vias: 190.04,79.28
N$1785  (via drill 0.8 pad 1.93)
  other vias: 190.04,76.74
N$1786  (via drill 0.8 pad 1.93)
  other vias: 190.04,74.2
N$1787  (via drill 0.8 pad 1.93)
  other vias: 190.04,71.66
N$1788  (via drill 0.8 pad 1.93)
  other vias: 190.04,69.12
N$1789  (via drill 0.8 pad 1.93)
  other vias: 190.04,66.58
N$1790  (via drill 0.8 pad 1.93)
  other vias: 190.04,64.04
N$1791  (via drill 0.8 pad 1.93)
  other vias: 190.04,61.5
N$1792  (via drill 0.8 pad 1.93)
  other vias: 190.04,58.96
N$1793  (via drill 0.8 pad 1.93)
  other vias: 190.04,56.42
N$1794  (via drill 0.8 pad 1.93)
  other vias: 190.04,53.88
N$1795  (via drill 0.8 pad 1.93)
  other vias: 190.04,51.34
N$1796  (via drill 0.8 pad 1.93)
  other vias: 190.04,48.8
N$1797  (via drill 0.8 pad 1.93)
  other vias: 190.04,46.26
N$1798  (via drill 0.8 pad 1.93)
  other vias: 190.04,43.72
N$1799  (via drill 0.8 pad 1.93)
  other vias: 190.04,41.18
N$1800  (via drill 0.8 pad 1.93)
  other vias: 190.04,38.64
N$1801  (via drill 0.8 pad 1.93)
  other vias: 190.04,36.1
N$1802  (via drill 0.8 pad 1.93)
  other vias: 190.04,33.56
N$1803  (via drill 0.8 pad 1.93)
  other vias: 190.04,31.02
N$1804  (via drill 0.8 pad 1.93)
  other vias: 190.04,28.48
N$1805  (via drill 0.8 pad 1.93)
  other vias: 190.04,25.94
N$1807  (via drill 0.8 pad 1.93)
  other vias: 192.58,119.92
N$1808  (via drill 0.8 pad 1.93)
  other vias: 192.58,117.38
N$1809  (via drill 0.8 pad 1.93)
  other vias: 192.58,114.84
N$1810  (via drill 0.8 pad 1.93)
  other vias: 192.58,112.3
N$1811  (via drill 0.8 pad 1.93)
  other vias: 192.58,109.76
N$1812  (via drill 0.8 pad 1.93)
  other vias: 192.58,107.22
N$1813  (via drill 0.8 pad 1.93)
  other vias: 192.58,104.68
N$1814  (via drill 0.8 pad 1.93)
  other vias: 192.58,102.14
N$1815  (via drill 0.8 pad 1.93)
  other vias: 192.58,99.6
N$1816  (via drill 0.8 pad 1.93)
  other vias: 192.58,97.06
N$1817  (via drill 0.8 pad 1.93)
  other vias: 192.58,94.52
N$1818  (via drill 0.8 pad 1.93)
  other vias: 192.58,91.98
N$1819  (via drill 0.8 pad 1.93)
  other vias: 192.58,89.44
N$1820  (via drill 0.8 pad 1.93)
  other vias: 192.58,86.9
N$1821  (via drill 0.8 pad 1.93)
  other vias: 192.58,84.36
N$1822  (via drill 0.8 pad 1.93)
  other vias: 192.58,81.82
N$1823  (via drill 0.8 pad 1.93)
  other vias: 192.58,79.28
N$1824  (via drill 0.8 pad 1.93)
  other vias: 192.58,76.74
N$1825  (via drill 0.8 pad 1.93)
  other vias: 192.58,74.2
N$1826  (via drill 0.8 pad 1.93)
  other vias: 192.58,71.66
N$1827  (via drill 0.8 pad 1.93)
  other vias: 192.58,69.12
N$1828  (via drill 0.8 pad 1.93)
  other vias: 192.58,66.58
N$1829  (via drill 0.8 pad 1.93)
  other vias: 192.58,64.04
N$1830  (via drill 0.8 pad 1.93)
  other vias: 192.58,61.5
N$1831  (via drill 0.8 pad 1.93)
  other vias: 192.58,58.96
N$1832  (via drill 0.8 pad 1.93)
  other vias: 192.58,56.42
N$1833  (via drill 0.8 pad 1.93)
  other vias: 192.58,53.88
N$1834  (via drill 0.8 pad 1.93)
  other vias: 192.58,51.34
N$1835  (via drill 0.8 pad 1.93)
  other vias: 192.58,48.8
N$1836  (via drill 0.8 pad 1.93)
  other vias: 192.58,46.26
N$1837  (via drill 0.8 pad 1.93)
  other vias: 192.58,43.72
N$1838  (via drill 0.8 pad 1.93)
  other vias: 192.58,41.18
N$1839  (via drill 0.8 pad 1.93)
  other vias: 192.58,38.64
N$1840  (via drill 0.8 pad 1.93)
  other vias: 192.58,36.1
N$1841  (via drill 0.8 pad 1.93)
  other vias: 192.58,33.56
N$1842  (via drill 0.8 pad 1.93)
  other vias: 192.58,31.02
N$1843  (via drill 0.8 pad 1.93)
  other vias: 192.58,28.48
N$1844  (via drill 0.8 pad 1.93)
  other vias: 192.58,25.94
N$1846  (via drill 0.8 pad 1.93)
  other vias: 195.12,119.92
N$1847  (via drill 0.8 pad 1.93)
  other vias: 195.12,117.38
N$1848  (via drill 0.8 pad 1.93)
  other vias: 195.12,114.84
N$1849  (via drill 0.8 pad 1.93)
  other vias: 195.12,112.3
N$1850  (via drill 0.8 pad 1.93)
  other vias: 195.12,109.76
N$1851  (via drill 0.8 pad 1.93)
  other vias: 195.12,107.22
N$1852  (via drill 0.8 pad 1.93)
  other vias: 195.12,104.68
N$1853  (via drill 0.8 pad 1.93)
  other vias: 195.12,102.14
N$1854  (via drill 0.8 pad 1.93)
  other vias: 195.12,99.6
N$1855  (via drill 0.8 pad 1.93)
  other vias: 195.12,97.06
N$1856  (via drill 0.8 pad 1.93)
  other vias: 195.12,94.52
N$1857  (via drill 0.8 pad 1.93)
  other vias: 195.12,91.98
N$1858  (via drill 0.8 pad 1.93)
  other vias: 195.12,89.44
N$1859  (via drill 0.8 pad 1.93)
  other vias: 195.12,86.9
N$1860  (via drill 0.8 pad 1.93)
  other vias: 195.12,84.36
N$1861  (via drill 0.8 pad 1.93)
  other vias: 195.12,81.82
N$1862  (via drill 0.8 pad 1.93)
  other vias: 195.12,79.28
N$1863  (via drill 0.8 pad 1.93)
  other vias: 195.12,76.74
N$1864  (via drill 0.8 pad 1.93)
  other vias: 195.12,74.2
N$1865  (via drill 0.8 pad 1.93)
  other vias: 195.12,71.66
N$1866  (via drill 0.8 pad 1.93)
  other vias: 195.12,69.12
N$1867  (via drill 0.8 pad 1.93)
  other vias: 195.12,66.58
N$1868  (via drill 0.8 pad 1.93)
  other vias: 195.12,64.04
N$1869  (via drill 0.8 pad 1.93)
  other vias: 195.12,61.5
N$1870  (via drill 0.8 pad 1.93)
  other vias: 195.12,58.96
N$1871  (via drill 0.8 pad 1.93)
  other vias: 195.12,56.42
N$1872  (via drill 0.8 pad 1.93)
  other vias: 195.12,53.88
N$1873  (via drill 0.8 pad 1.93)
  other vias: 195.12,51.34
N$1874  (via drill 0.8 pad 1.93)
  other vias: 195.12,48.8
N$1875  (via drill 0.8 pad 1.93)
  other vias: 195.12,46.26
N$1876  (via drill 0.8 pad 1.93)
  other vias: 195.12,43.72
N$1877  (via drill 0.8 pad 1.93)
  other vias: 195.12,41.18
N$1878  (via drill 0.8 pad 1.93)
  other vias: 195.12,38.64
N$1879  (via drill 0.8 pad 1.93)
  other vias: 195.12,36.1
N$1880  (via drill 0.8 pad 1.93)
  other vias: 195.12,33.56
N$1881  (via drill 0.8 pad 1.93)
  other vias: 195.12,31.02
N$1882  (via drill 0.8 pad 1.93)
  other vias: 195.12,28.48
N$1883  (via drill 0.8 pad 1.93)
  other vias: 195.12,25.94
N$1885  (via drill 0.8 pad 1.93)
  other vias: 197.66,119.92
N$1886  (via drill 0.8 pad 1.93)
  other vias: 197.66,117.38
N$1887  (via drill 0.8 pad 1.93)
  other vias: 197.66,114.84
N$1888  (via drill 0.8 pad 1.93)
  other vias: 197.66,112.3
N$1889  (via drill 0.8 pad 1.93)
  other vias: 197.66,109.76
N$1890  (via drill 0.8 pad 1.93)
  other vias: 197.66,107.22
N$1891  (via drill 0.8 pad 1.93)
  other vias: 197.66,104.68
N$1892  (via drill 0.8 pad 1.93)
  other vias: 197.66,102.14
N$1893  (via drill 0.8 pad 1.93)
  other vias: 197.66,99.6
N$1894  (via drill 0.8 pad 1.93)
  other vias: 197.66,97.06
N$1895  (via drill 0.8 pad 1.93)
  other vias: 197.66,94.52
N$1896  (via drill 0.8 pad 1.93)
  other vias: 197.66,91.98
N$1897  (via drill 0.8 pad 1.93)
  other vias: 197.66,89.44
N$1898  (via drill 0.8 pad 1.93)
  other vias: 197.66,86.9
N$1899  (via drill 0.8 pad 1.93)
  other vias: 197.66,84.36
N$1900  (via drill 0.8 pad 1.93)
  other vias: 197.66,81.82
N$1901  (via drill 0.8 pad 1.93)
  other vias: 197.66,79.28
N$1902  (via drill 0.8 pad 1.93)
  other vias: 197.66,76.74
N$1903  (via drill 0.8 pad 1.93)
  other vias: 197.66,74.2
N$1904  (via drill 0.8 pad 1.93)
  other vias: 197.66,71.66
N$1905  (via drill 0.8 pad 1.93)
  other vias: 197.66,69.12
N$1906  (via drill 0.8 pad 1.93)
  other vias: 197.66,66.58
N$1907  (via drill 0.8 pad 1.93)
  other vias: 197.66,64.04
N$1908  (via drill 0.8 pad 1.93)
  other vias: 197.66,61.5
N$1909  (via drill 0.8 pad 1.93)
  other vias: 197.66,58.96
N$1910  (via drill 0.8 pad 1.93)
  other vias: 197.66,56.42
N$1911  (via drill 0.8 pad 1.93)
  other vias: 197.66,53.88
N$1912  (via drill 0.8 pad 1.93)
  other vias: 197.66,51.34
N$1913  (via drill 0.8 pad 1.93)
  other vias: 197.66,48.8
N$1914  (via drill 0.8 pad 1.93)
  other vias: 197.66,46.26
N$1915  (via drill 0.8 pad 1.93)
  other vias: 197.66,43.72
N$1916  (via drill 0.8 pad 1.93)
  other vias: 197.66,41.18
N$1917  (via drill 0.8 pad 1.93)
  other vias: 197.66,38.64
N$1918  (via drill 0.8 pad 1.93)
  other vias: 197.66,36.1
N$1919  (via drill 0.8 pad 1.93)
  other vias: 197.66,33.56
N$1920  (via drill 0.8 pad 1.93)
  other vias: 197.66,31.02
N$1921  (via drill 0.8 pad 1.93)
  other vias: 197.66,28.48
N$1922  (via drill 0.8 pad 1.93)
  other vias: 197.66,25.94
N$1924  (via drill 0.8 pad 1.93)
  other vias: 200.2,119.92
N$1925  (via drill 0.8 pad 1.93)
  other vias: 200.2,117.38
N$1926  (via drill 0.8 pad 1.93)
  other vias: 200.2,114.84
N$1927  (via drill 0.8 pad 1.93)
  other vias: 200.2,112.3
N$1928  (via drill 0.8 pad 1.93)
  other vias: 200.2,109.76
N$1929  (via drill 0.8 pad 1.93)
  other vias: 200.2,107.22
N$1930  (via drill 0.8 pad 1.93)
  other vias: 200.2,104.68
N$1931  (via drill 0.8 pad 1.93)
  other vias: 200.2,102.14
N$1932  (via drill 0.8 pad 1.93)
  other vias: 200.2,99.6
N$1933  (via drill 0.8 pad 1.93)
  other vias: 200.2,97.06
N$1934  (via drill 0.8 pad 1.93)
  other vias: 200.2,94.52
N$1935  (via drill 0.8 pad 1.93)
  other vias: 200.2,91.98
N$1936  (via drill 0.8 pad 1.93)
  other vias: 200.2,89.44
N$1937  (via drill 0.8 pad 1.93)
  other vias: 200.2,86.9
N$1938  (via drill 0.8 pad 1.93)
  other vias: 200.2,84.36
N$1939  (via drill 0.8 pad 1.93)
  other vias: 200.2,81.82
N$1940  (via drill 0.8 pad 1.93)
  other vias: 200.2,79.28
N$1941  (via drill 0.8 pad 1.93)
  other vias: 200.2,76.74
N$1942  (via drill 0.8 pad 1.93)
  other vias: 200.2,74.2
N$1943  (via drill 0.8 pad 1.93)
  other vias: 200.2,71.66
N$1944  (via drill 0.8 pad 1.93)
  other vias: 200.2,69.12
N$1945  (via drill 0.8 pad 1.93)
  other vias: 200.2,66.58
N$1946  (via drill 0.8 pad 1.93)
  other vias: 200.2,64.04
N$1947  (via drill 0.8 pad 1.93)
  other vias: 200.2,61.5
N$1948  (via drill 0.8 pad 1.93)
  other vias: 200.2,58.96
N$1949  (via drill 0.8 pad 1.93)
  other vias: 200.2,56.42
N$1950  (via drill 0.8 pad 1.93)
  other vias: 200.2,53.88
N$1951  (via drill 0.8 pad 1.93)
  other vias: 200.2,51.34
N$1952  (via drill 0.8 pad 1.93)
  other vias: 200.2,48.8
N$1953  (via drill 0.8 pad 1.93)
  other vias: 200.2,46.26
N$1954  (via drill 0.8 pad 1.93)
  other vias: 200.2,43.72
N$1955  (via drill 0.8 pad 1.93)
  other vias: 200.2,41.18
N$1956  (via drill 0.8 pad 1.93)
  other vias: 200.2,38.64
N$1957  (via drill 0.8 pad 1.93)
  other vias: 200.2,36.1
N$1958  (via drill 0.8 pad 1.93)
  other vias: 200.2,33.56
N$1959  (via drill 0.8 pad 1.93)
  other vias: 200.2,31.02
N$1960  (via drill 0.8 pad 1.93)
  other vias: 200.2,28.48
N$1961  (via drill 0.8 pad 1.93)
  other vias: 200.2,25.94
N$1964  (via drill 0.8 pad 1.93)
  other vias: 202.74,117.38
N$1965  (via drill 0.8 pad 1.93)
  other vias: 202.74,114.84
N$1966  (via drill 0.8 pad 1.93)
  other vias: 202.74,112.3
N$1967  (via drill 0.8 pad 1.93)
  other vias: 202.74,109.76
N$1968  (via drill 0.8 pad 1.93)
  other vias: 202.74,107.22
N$1969  (via drill 0.8 pad 1.93)
  other vias: 202.74,104.68
N$1970  (via drill 0.8 pad 1.93)
  other vias: 202.74,102.14
N$1971  (via drill 0.8 pad 1.93)
  other vias: 202.74,99.6
N$1972  (via drill 0.8 pad 1.93)
  other vias: 202.74,97.06
N$1973  (via drill 0.8 pad 1.93)
  other vias: 202.74,94.52
N$1974  (via drill 0.8 pad 1.93)
  other vias: 202.74,91.98
N$1975  (via drill 0.8 pad 1.93)
  other vias: 202.74,89.44
N$1976  (via drill 0.8 pad 1.93)
  other vias: 202.74,86.9
N$1977  (via drill 0.8 pad 1.93)
  other vias: 202.74,84.36
N$1978  (via drill 0.8 pad 1.93)
  other vias: 202.74,81.82
N$1979  (via drill 0.8 pad 1.93)
  other vias: 202.74,79.28
N$1980  (via drill 0.8 pad 1.93)
  other vias: 202.74,76.74
N$1981  (via drill 0.8 pad 1.93)
  other vias: 202.74,74.2
N$1982  (via drill 0.8 pad 1.93)
  other vias: 202.74,71.66
N$1983  (via drill 0.8 pad 1.93)
  other vias: 202.74,69.12
N$1984  (via drill 0.8 pad 1.93)
  other vias: 202.74,66.58
N$1985  (via drill 0.8 pad 1.93)
  other vias: 202.74,64.04
N$1986  (via drill 0.8 pad 1.93)
  other vias: 202.74,61.5
N$1987  (via drill 0.8 pad 1.93)
  other vias: 202.74,58.96
N$1988  (via drill 0.8 pad 1.93)
  other vias: 202.74,56.42
N$1989  (via drill 0.8 pad 1.93)
  other vias: 202.74,53.88
N$1990  (via drill 0.8 pad 1.93)
  other vias: 202.74,51.34
N$1991  (via drill 0.8 pad 1.93)
  other vias: 202.74,48.8
N$1992  (via drill 0.8 pad 1.93)
  other vias: 202.74,46.26
N$1993  (via drill 0.8 pad 1.93)
  other vias: 202.74,43.72
N$1994  (via drill 0.8 pad 1.93)
  other vias: 202.74,41.18
N$1995  (via drill 0.8 pad 1.93)
  other vias: 202.74,38.64
N$1996  (via drill 0.8 pad 1.93)
  other vias: 202.74,36.1
N$1997  (via drill 0.8 pad 1.93)
  other vias: 202.74,33.56
N$1998  (via drill 0.8 pad 1.93)
  other vias: 202.74,31.02
N$1999  (via drill 0.8 pad 1.93)
  other vias: 202.74,28.48
N$2004  (via drill 0.8 pad 1.93)
  other vias: 205.28,114.84
N$2005  (via drill 0.8 pad 1.93)
  other vias: 205.28,112.3
N$2006  (via drill 0.8 pad 1.93)
  other vias: 205.28,109.76
N$2007  (via drill 0.8 pad 1.93)
  other vias: 205.28,107.22
N$2008  (via drill 0.8 pad 1.93)
  other vias: 205.28,104.68
N$2009  (via drill 0.8 pad 1.93)
  other vias: 205.28,102.14
N$2010  (via drill 0.8 pad 1.93)
  other vias: 205.28,99.6
N$2011  (via drill 0.8 pad 1.93)
  other vias: 205.28,97.06
N$2012  (via drill 0.8 pad 1.93)
  other vias: 205.28,94.52
N$2013  (via drill 0.8 pad 1.93)
  other vias: 205.28,91.98
N$2014  (via drill 0.8 pad 1.93)
  other vias: 205.28,89.44
N$2015  (via drill 0.8 pad 1.93)
  other vias: 205.28,86.9
N$2016  (via drill 0.8 pad 1.93)
  other vias: 205.28,84.36
N$2017  (via drill 0.8 pad 1.93)
  other vias: 205.28,81.82
N$2018  (via drill 0.8 pad 1.93)
  other vias: 205.28,79.28
N$2019  (via drill 0.8 pad 1.93)
  other vias: 205.28,76.74
N$2020  (via drill 0.8 pad 1.93)
  other vias: 205.28,74.2
N$2021  (via drill 0.8 pad 1.93)
  other vias: 205.28,71.66
N$2022  (via drill 0.8 pad 1.93)
  other vias: 205.28,69.12
N$2023  (via drill 0.8 pad 1.93)
  other vias: 205.28,66.58
N$2024  (via drill 0.8 pad 1.93)
  other vias: 205.28,64.04
N$2025  (via drill 0.8 pad 1.93)
  other vias: 205.28,61.5
N$2026  (via drill 0.8 pad 1.93)
  other vias: 205.28,58.96
N$2027  (via drill 0.8 pad 1.93)
  other vias: 205.28,56.42
N$2028  (via drill 0.8 pad 1.93)
  other vias: 205.28,53.88
N$2029  (via drill 0.8 pad 1.93)
  other vias: 205.28,51.34
N$2030  (via drill 0.8 pad 1.93)
  other vias: 205.28,48.8
N$2031  (via drill 0.8 pad 1.93)
  other vias: 205.28,46.26
N$2032  (via drill 0.8 pad 1.93)
  other vias: 205.28,43.72
N$2033  (via drill 0.8 pad 1.93)
  other vias: 205.28,41.18
N$2034  (via drill 0.8 pad 1.93)
  other vias: 205.28,38.64
N$2035  (via drill 0.8 pad 1.93)
  other vias: 205.28,36.1
N$2036  (via drill 0.8 pad 1.93)
  other vias: 205.28,33.56
N$2037  (via drill 0.8 pad 1.93)
  other vias: 205.28,31.02

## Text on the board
bPlace: AB5HM | Hermes Lite TRX V1.0
tNames: UM + G - | +12V | GND | MIC pre amp | AB5HM
bNames: + | GND | 1 | + | GND | 1 | 1 | PTT | 1 | 1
